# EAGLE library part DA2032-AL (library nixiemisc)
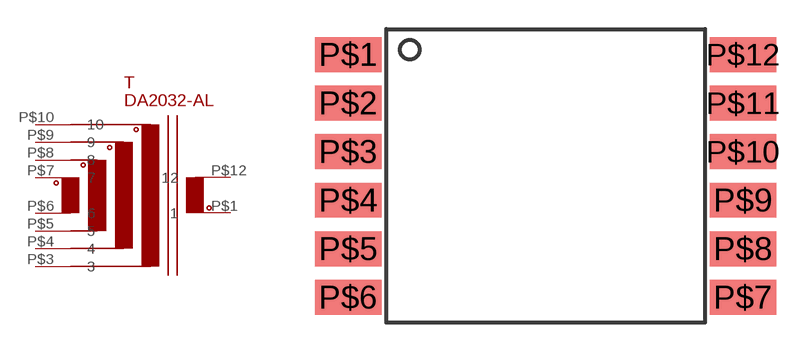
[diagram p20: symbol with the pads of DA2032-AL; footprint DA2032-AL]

Designator prefix T

## DA2032-AL  [DA2032-AL]
P$1  1  pas
P$3  3  pas
P$4  4  pas
P$5  5  pas
P$6  6  pas
P$7  7  pas
P$8  8  pas
P$9  9  pas
P$10  10  pas
P$12  12  pas

## Footprint DA2032-AL (pad centres in mm)
smd 3.43 x 1.79: P$1 -10.155,6.25; P$2 -10.155,3.75; P$3 -10.155,1.25; P$4 -10.155,-1.25; P$5 -10.155,-3.75; P$6 -10.155,-6.25; P$7 10.155,-6.25; P$8 10.155,-3.75; P$9 10.155,-1.25; P$10 10.155,1.25; P$11 10.155,3.75; P$12 10.155,6.25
